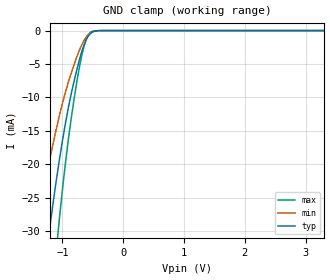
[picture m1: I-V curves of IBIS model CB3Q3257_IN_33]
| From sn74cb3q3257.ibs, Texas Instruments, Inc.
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[Model]   CB3Q3257_IN_33
Model_type  Input
Vinl=0.8
Vinh=2.0
| variable   typ   min   max
C_comp   2.91pF   2.24pF   4.29pF
[Temperature Range]   40   100   -40
| Ambient temperature   25   85   -40
[Voltage range]   3.3   3   3.6
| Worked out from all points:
|   GND clamp passes 1 mA (typ) near -0.59 V on its own axis
[GND Clamp]
| CB3Q3257_IN_33
|   Voltage   I(typ)   I(min)   I(max)
-5.5V     -472.4mA   -358mA     -596.1mA
-1.43V    -45.98mA   -30.17mA   -67.32mA
-1.22V    -30.26mA   -19.79mA   -44.58mA
-1.08V    -21.12mA   -13.88mA   -30.89mA
-1.06V    -19.92mA   -13.1mA    -29.06mA
-975mV    -15.15mA   -10.04mA   -21.76mA
-900mV    -11.44mA   -7.635mA   -16.11mA
-770mV    -6.108mA   -4.099mA   -8.049mA
-645mV    -2.181mA   -1.479mA   -2.339mA
-535mV    -406.2uA   -314.8uA   -251uA
-330mV    -2.055uA   -3.329uA   -188.5nA
3.3V      128.8pA    501.8pA    26.94pA
